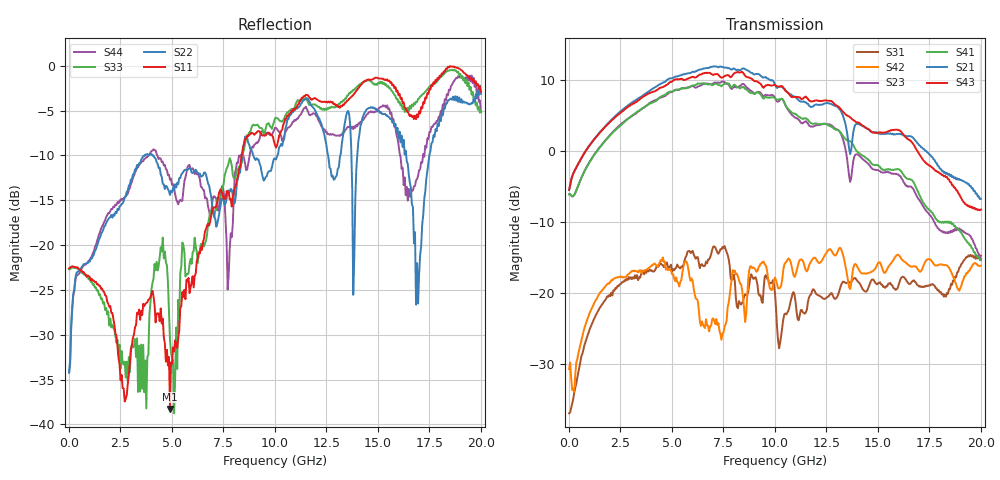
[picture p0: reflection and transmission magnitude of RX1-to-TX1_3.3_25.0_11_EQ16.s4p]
!Agilent Technologies,N5225A,MY51451112,A.09.50.13
!Agilent N5225A: A.09.50.13
!Date: Wednesday, January 31, 2018 11:06:30
!Correction: S11(Full 4 Port(1,2,3,4))
!S12(Full 4 Port(1,2,3,4))
!S13(Full 4 Port(1,2,3,4))
!S14(Full 4 Port(1,2,3,4))
!S21(Full 4 Port(1,2,3,4))
!S22(Full 4 Port(1,2,3,4))
!S23(Full 4 Port(1,2,3,4))
!S24(Full 4 Port(1,2,3,4))
!S31(Full 4 Port(1,2,3,4))
!S32(Full 4 Port(1,2,3,4))
!S33(Full 4 Port(1,2,3,4))
!S34(Full 4 Port(1,2,3,4))
!S41(Full 4 Port(1,2,3,4))
!S42(Full 4 Port(1,2,3,4))
!S43(Full 4 Port(1,2,3,4))
!S44(Full 4 Port(1,2,3,4))
!S4P File: Measurements: <S11,S12,S13,S14>,
!<S21,S22,S23,S24>,
!<S31,S32,S33,S34>,
!<S41,S42,S43,S44>:
# Hz S  RI  R 50
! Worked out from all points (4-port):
!   401 points, 10 MHz to 20 GHz, reference 50 ohm
!   strongest paths, dB at 10 MHz, 5.008 GHz, 10.01 GHz, 15 GHz, 20 GHz:
!     S43: -5.5, 9.8, 9.4, 2.6, -8.2
!     S21: -5.4, 10.3, 9.4, 2.6, -6.7
!     S41: -6.1, 8.4, 7.5, -1.9, -15.4
!     S23: -6.1, 8.3, 7.6, -2.7, -15.2
!     S42: -30.7, -17.3, -17.8, -15.8, -16.1
!     S31: -36.9, -17.0, -20.1, -18.6, -14.7
!   lowest |S11| = -38.3 dB at 4.908 GHz (marker M1), VSWR 1.02, Z = 50.1 - j1.22 ohm
!   |S11| at or under -10 dB: start of sweep to 8.391 GHz
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1e7  -0.0742 -0.0031  -0.000265 0.000685  0.0139 0.000477  -1.47e-05 0.000377
     0.5356 0.0155  -0.0136 0.014  -0.4975 -0.00376  0.0266 0.0122
     0.0142 0.000795  0.000197 0.000475  -0.0733 -0.00374  -0.000179 0.000459
     -0.4979 -0.00333  0.0265 0.0122  0.5337 0.0146  -0.0129 0.0145
2.70865e9  -0.00916 -0.0098  0.0158 0.00347  0.0518 0.1118  0.0175 0.000764
           1.69 -1.107  0.1833 0.0166  -1.316 0.9655  0.1013 0.092
           0.0596 0.1082  0.019 0.00403  0.00403 0.022  0.021 0.000781
           -1.16 1.122  0.0871 0.0955  1.383 -1.404  0.1821 -0.0329
4.90755e9  0.00123 -0.0121  0.0188 0.000319  0.1071 0.1086  0.018 -0.00887
           -0.9939 -3.108  0.169 -0.0866  1.097 2.37  0.1285 0.0364
           0.1041 0.1136  0.0167 -0.00349  0.0162 -0.0246  0.0151 -0.00948
           1.728 1.984  0.1442 0.0155  -1.854 -2.448  0.1334 -0.1889
6.956525e9  -0.034 0.1526  0.0133 -0.0153  0.1393 0.0509  0.0106 -0.0268
            -3.887 0.6144  0.1026 -0.1307  2.839 -0.8977  0.0231 0.0371
            0.1541 0.1309  0.0203 -0.0139  0.0238 0.1491  0.0236 -0.0306
            2.181 -1.938  0.0647 -0.0108  -2.744 2.133  0.0913 -0.1455
8.555725e9  -0.00925 0.3913  -0.00329 -0.0103  0.0624 0.021  -0.00271 -0.0158
            -0.7099 3.718  -0.1473 0.3754  0.0116 -2.897  -0.0202 0.1254
            0.0876 0.0441  0.00768 -0.0128  0.0159 0.3731  -0.00114 -0.0336
            -1.236 -2.458  0.00158 0.0626  1.26 3.158  0.2205 0.1776
1.250375e10  0.2374 0.5847  -0.0323 -0.0165  0.0108 0.0916  -0.0275 0.00332
             1.815 -1.215  0.1626 0.319  -0.9984 1.193  0.177 0.0903
             0.0225 0.0899  -0.0251 -0.0158  0.3356 0.457  -0.0306 -0.00954
             -0.0275 1.549  0.1599 0.1071  0.3672 -2.245  0.3089 -0.2984
2e10  0.7119 0.0742  0.023 0.0349  -0.0811 0.1568  0.0349 0.0208
      0.0821 0.4548  0.6935 0.0746  -0.0466 -0.1679  0.1556 0.0385
      -0.0786 0.166  0.00619 0.048  0.5631 -0.0216  0.0475 0.0206
      -0.1701 -0.0106  0.1492 0.0454  0.381 0.0722  -0.151 -0.5312
